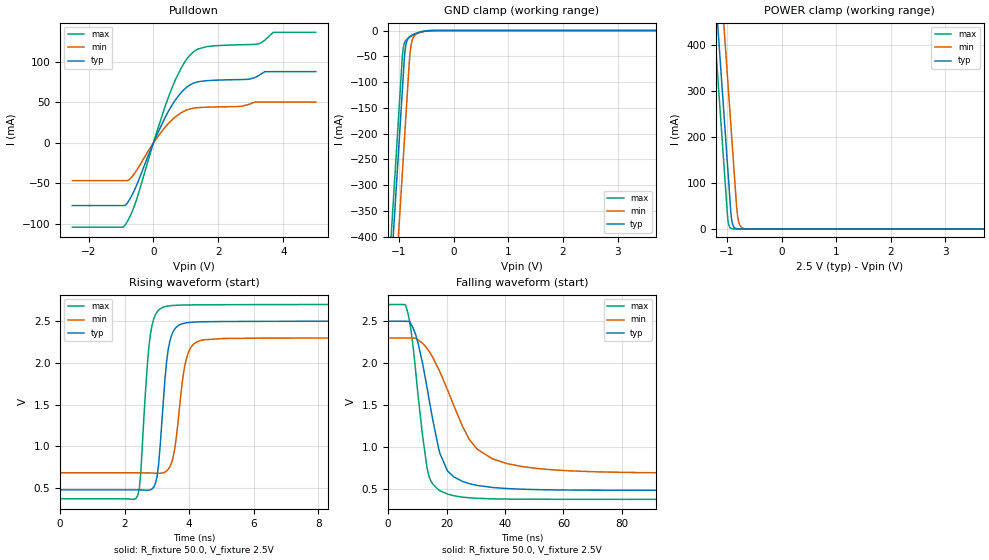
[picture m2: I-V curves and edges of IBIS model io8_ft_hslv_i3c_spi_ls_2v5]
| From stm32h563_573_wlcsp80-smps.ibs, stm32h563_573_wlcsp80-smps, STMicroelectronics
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[Model]   io8_ft_hslv_i3c_spi_ls_2v5
Model_type I/O_open_drain
Polarity   Non-Inverting
Enable   Active-Low
| CAP_THRESHOLD on pad IOFT is "UDTCAPC" :
| Rising=20.0% of vddiom   Falling=80.0% of vddiom
| C_comp min and max val. don't necessarily correlate with the min and max pvt
| but are the smallest and greatest pad capacitance found.
| var   typ   min   max
C_comp   3.87198pF  3.86881pF  3.96694pF
|C_comp_pulldown   3.87198pF  3.86881pF  3.96694pF
Vinl = 1.15V
Vinh = 1.35V
Vmeas = 1.25V   | Reference voltage for timing measurements
Cref  = 50.0pF   | Timing specification test load capacitance value
Rref  = 1.0MOhm   | Timing specification test load resistance value
Vref  = 1.375V   | Timing specification test load voltage
[Model Spec]
| TIME_THRESHOLD on pin ZII2CV11 is "CMOS" :
| Rising=40.0% of vdd   Falling=60.0% of vdd
Vinl 989.80000mV 917.80000mV 1.06580V
Vinh 1.40320V 1.29620V 1.49120V
| variable   typ   min   max
[Temperature Range] 25.0 125.0 -40.0
| variable   typ   min   max
[Voltage Range] 2.5V 2.3V 2.7V
| variable   typ   min   max
[POWER Clamp Reference] 2.5V 2.3V 2.7V
| variable   typ   min   max
[GND Clamp Reference] 0V 0V 0V
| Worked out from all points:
|   slope of the pulldown table from 0 to 0.375 V, typ, clamps not added: 11.5 ohm
|   GND clamp passes 1 mA (typ) near -0.52 V on its own axis
|   POWER clamp passes 1 mA (typ) near -0.84 V on its own axis
|   rising waveform, R_fixture 50.0, V_fixture 2.5V: 20-80 % time 254ps typ, 306ps min, 242ps max; typ from 0.481 V to 2.5 V
|   falling waveform, R_fixture 50.0, V_fixture 2.5V: 20-80 % time 7.01ns typ, 13.1ns min, 4.54ns max; typ from 2.5 V to 0.481 V
[POWER Clamp]
-2.5V     2.708A     2.899A     2.597A
-1.23V    548.8mA    740.2mA    437.5mA
-1.16V    429.8mA    621.2mA    318.5mA
-1.12V    361.8mA    553.2mA    250.5mA
-1.03V    208.8mA    400.2mA    97.53mA
-980mV    123.8mA    315.2mA    17.95mA
-920mV    26.3mA     213.2mA    906uA
-880mV    5.543mA    145.2mA    123.7uA
-810mV    363.5uA    33.6mA     3.797uA
-770mV    76.62uA    10.47mA    518.8nA
-700mV    5.026uA    1.361mA    16.11nA
5V        0A         0A         0A
[GND Clamp]
-2.5V     -2.77A     -2.931A    -2.704A
-1.21V    -576.8mA   -738.1mA   -511.3mA
-950mV    -134.8mA   -296.1mA   -69.34mA
-920mV    -83.82mA   -245.1mA   -32.48mA
-900mV    -50.56mA   -211.1mA   -24.02mA
-880mV    -31.31mA   -177.1mA   -19.85mA
-850mV    -18.7mA    -126.1mA   -16.34mA
-800mV    -11.46mA   -46.18mA   -12.45mA
-750mV    -8.203mA   -16.63mA   -9.325mA
-650mV    -4.063mA   -4.987mA   -4.427mA
-360mV    -35.05uA   -165.1uA   -9.564uA
5V        7.96nA     1.281uA    294pA
| variable   typ   min   max
[Pullup Reference] 2.5V 2.3V 2.7V
| variable   typ   min   max
[Pulldown Reference] 0V 0V 0V
[Pulldown]
-2.5V     -77.63mA   -46.85mA   -104.3mA
-870mV    -77.24mA   -46.85mA   -101.4mA
-550mV    -55.3mA    -35.88mA   -73.72mA
90mV      8.401mA    5.299mA    11.79mA
610mV     49.03mA    29.75mA    71.69mA
870mV     62.92mA    37.48mA    93.62mA
1.23V     73.63mA    42.72mA    112.2mA
1.64V     76.78mA    44.01mA    118.8mA
2.7V      78.15mA    44.99mA    121.2mA
3.22V     82.58mA    50.35mA    122.2mA
3.69V     87.93mA    50.35mA    136.5mA
5V        87.93mA    50.35mA    136.5mA
[Ramp]
dV/dt_r 1.21163V/249.73748ps 969.23227mV/302.37887ps 1.39627V/238.7333ps
dV/dt_f 1.21165V/6.77877ns 969.25317mV/12.85645ns 1.39628V/4.50418ns
R_load = 50.0
| Removed startup time: 0s 0s 0s  .
| Removed end time: 49.4ns.
[Rising Waveform]
R_fixture   = 50.0
V_fixture   = 2.5V
V_fixture_min = 2.3V
V_fixture_max = 2.7V
0s        480.6mV    684.6mV    372.9mV
2.4ns     480.4mV    684.7mV    408.7mV
2.5ns     479.9mV    684.6mV    688.1mV
2.8ns     481.4mV    683mV      2.348V
3.05ns    775.7mV    678.2mV    2.632V
3.25ns    1.812V     693.1mV    2.674V
3.4ns     2.26V      757mV      2.685V
3.9ns     2.48V      2.032V     2.694V
4.45ns    2.493V     2.277V     2.696V
49.4ns    2.5V       2.3V       2.7V
| Removed startup time: 0s 0s 0s  .
| Removed end time: 249.4ns.
[Falling Waveform]
R_fixture   = 50.0
V_fixture   = 2.5V
V_fixture_min = 2.3V
V_fixture_max = 2.7V
0s        2.5V       2.3V       2.7V
5.95ns    2.5V       2.3V       2.696V
8.6ns     2.417V     2.299V     2.183V
11.75ns   2.008V     2.239V     1.15V
13.65ns   1.644V     2.16V      696mV
17.7ns    923.5mV    1.898V     476.5mV
20.35ns   710.6mV    1.68V      435.5mV
30.55ns   538.7mV    969.8mV    384.8mV
50.9ns    489.1mV    741.7mV    373.7mV
249.4ns   480.6mV    684.6mV    372.9mV
